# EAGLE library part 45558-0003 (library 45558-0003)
MOLEX - 45558-0003 - CONNECTOR, HEADER, 6POS, 2ROW, 4.2MM Source: Datasheet
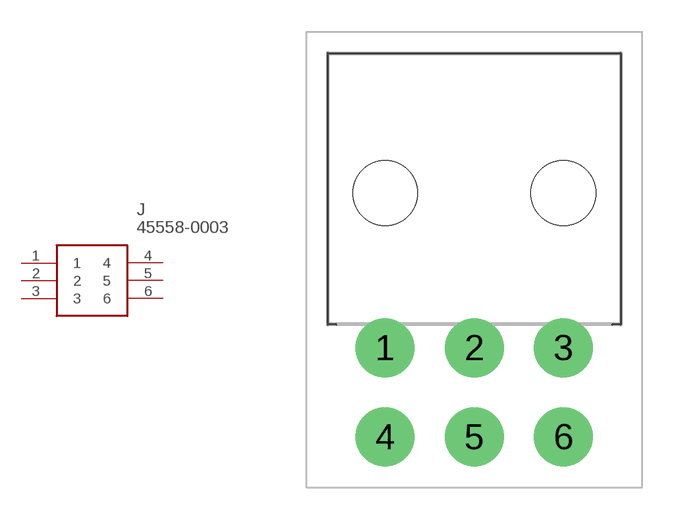
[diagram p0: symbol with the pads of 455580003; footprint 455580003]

Designator prefix J

## 45558-0003 (Allied_Number: 71464452; Allied_Price-Stock: https://www.alliedelec.com/molexincorporated-45558-0003/71464452/; Description: MOLEX - 45558-0003 - CONNECTOR, HEADER, 6POS, 2ROW, 4.2MM; Height: 10mm; Manufacturer_Name: Molex; Manufacturer_Part_Number: 45558-0003; Mouser_Part_Number: 538-45558-0003; Mouser_Price-Stock: https://www.mouser.com/Search/Refine.aspx?Keyword=538-45558-0003)  [455580003]
1  1
2  2
3  3
4  4
5  5
6  6

## Footprint 455580003 (pad centres in mm)
45558-0003-3
drill 1.85 pad 2.775: 1 0,0; 2 4.2,0; 3 8.4,0; 4 0,-4.2; 5 4.2,-4.2; 6 8.4,-4.2
hole 3.05 at 0,7.3
hole 3.05 at 8.4,7.3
